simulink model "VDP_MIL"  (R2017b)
settings: Solver=FixedStepDiscrete  StartTime=0.0  StopTime=10.0  FixedStep=0.01  RelTol=1e-3  EnableMultiTasking=on
undefined symbols (not defined in the file): ASWTYPE_FALSE, ASWTYPE_TRUE, CcVDP_DiagPermitDelayTi_ms, CcVDP_Kl30VoltNorm2Over_mV, CcVDP_Kl30VoltNorm2Under_mV, CcVDP_Kl30VoltOver2Norm_mV, CcVDP_Kl30VoltUnder2Norm_mV, CcVDP_LeadAcidChgHvOnTi_ms, VDP0B5_RUNTIME_MS, VDP2A3_RUNTIME_MS, VDP_CONST2080_NUMB
libraries: AIWAYS_Powertrain_BMS_lib x36

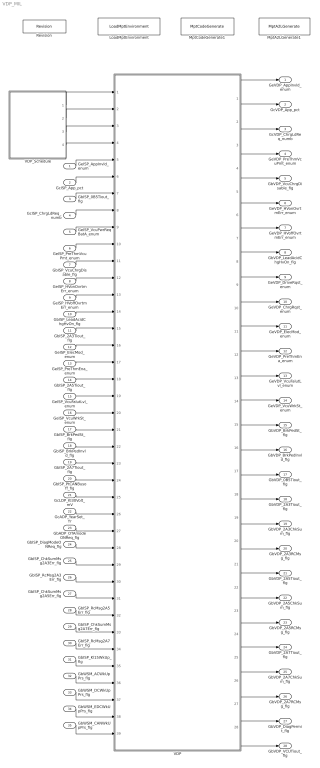
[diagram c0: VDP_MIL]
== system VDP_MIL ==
  GeISP_AppInvld_enum : Inport
  GcISP_App_pct : Inport  Port=2
  GbISP_0B5Tiout_flg : Inport  Port=3
  GcISP_ChrgLdReq_numb : Inport  Port=4
  GeISP_VcuPwrReqBatA_enum : Inport  Port=5
  GeISP_PreThmVcuPmt_enum : Inport  Port=6
  GbISP_VcuChrgDisable_flg : Inport  Port=7
  GeISP_HVonOvrtmErr_enum : Inport  Port=8
  GeISP_HVoffOvrtmErr_enum : Inport  Port=9
  GbISP_LeadAcidChgHvOn_flg : Inport  Port=10
  GbISP_2A3Tiout_flg : Inport  Port=11
  GeISP_ElecMod_enum : Inport  Port=12
  GeISP_PreThmEna_enum : Inport  Port=13
  GbISP_2A5Tiout_flg : Inport  Port=14
  GeISP_VcuFalutLvl_enum : Inport  Port=15
  GeISP_VcuWrkSt_enum : Inport  Port=16
  GbISP_BrkPedSt_flg : Inport  Port=17
  GbISP_BrkPedInvld_flg : Inport  Port=18
  GbISP_2A7Tiout_flg : Inport  Port=19
  GbISP_PtCANBusoff_flg : Inport  Port=20
  GcLDP_Kl30Volt_mV : Inport  Port=21
  GcADP_YearSet_Yr : Inport  Port=22
  GbADP_OTAmodeONReq_flg : Inport  Port=23
  GbISP_DiagModeONReq_flg : Inport  Port=24
  GbISP_ChkSumMsg2A3Err_flg : Inport  Port=25
  GbISP_RcMsg2A3Err_flg : Inport  Port=26
  GbISP_ChkSumMsg2A5Err_flg : Inport  Port=27
  GbISP_RcMsg2A5Err_flg : Inport  Port=28
  GbISP_ChkSumMsg2A7Err_flg : Inport  Port=29
  GbISP_RcMsg2A7Err_flg : Inport  Port=30
  GbISP_Kl15WkUp_flg : Inport  Port=31
  GbWSM_ACWkUpPrs_flg : Inport  Port=32
  GbWSM_DCWkUpPrs_flg : Inport  Port=33
  GbWSM_EDCWkUpPrs_flg : Inport  Port=34
  GbWSM_CANWkUpPrs_flg : Inport  Port=35
  LoadMptEnvironment : AIWAYS_Powertrain_BMS_lib/Config/LoadMptEnvironment  ProjectName=Comm  SuppierID=NewPlatformUAES
  MptA2LGenerate1 : AIWAYS_Powertrain_BMS_lib/Config/MptA2LGenerate  SystemSampleTime=-1
  MptCodeGenerate1 : AIWAYS_Powertrain_BMS_lib/Config/MptCodeGenerate  SystemSampleTime=-1
  Revision : AIWAYS_Powertrain_BMS_lib/Config/Revision  curVersion='M107C106'  newVersion='M107C106'
  VDP : Subsystem
  VDP_Schedule : Stateflow chart  TreatAsAtomicUnit=on
  GeVDP_AppInvld_enum : Outport
  GcVDP_App_pct : Outport  Port=2
  GcVDP_ChrgLdReq_numb : Outport  Port=3
  GeVDP_PreThmVcuPmt_enum : Outport  Port=4
  GbVDP_VcuChrgDisable_flg : Outport  Port=5
  GeVDP_HVonOvrtmErr_enum : Outport  Port=6
  GeVDP_HVoffOvrtmErr_enum : Outport  Port=7
  GbVDP_LeadAcidChgHvOn_flg : Outport  Port=8
  GeVDP_DriveRqst_enum : Outport  Port=9
  GeVDP_ChrgRqst_enum : Outport  Port=10
  GeVDP_ElecMod_enum : Outport  Port=11
  GeVDP_PreThmEna_enum : Outport  Port=12
  GeVDP_VcuFalutLvl_enum : Outport  Port=13
  GeVDP_VcuWrkSt_enum : Outport  Port=14
  GbVDP_BrkPedSt_flg : Outport  Port=15
  GbVDP_BrkPedInvld_flg : Outport  Port=16
  GbVDP_0B5Tiout_flg : Outport  Port=17
  GbVDP_2A3Tiout_flg : Outport  Port=18
  GbVDP_2A3ChkSum_flg : Outport  Port=19
  GbVDP_2A3RCMsg_flg : Outport  Port=20
  GbVDP_2A5Tiout_flg : Outport  Port=21
  GbVDP_2A5ChkSum_flg : Outport  Port=22
  GbVDP_2A5RCMsg_flg : Outport  Port=23
  GbVDP_2A7Tiout_flg : Outport  Port=24
  GbVDP_2A7ChkSum_flg : Outport  Port=25
  GbVDP_2A7RCMsg_flg : Outport  Port=26
  GbVDP_DiagPermit_flg : Outport  Port=27
  GbVDP_VCUTiout_flg : Outport  Port=28
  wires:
  GeISP_AppInvld_enum/1 -> VDP/5(GeISP_AppInvld_enum)
  GcISP_App_pct/1 -> VDP/6(GcISP_App_pct)
  GbISP_0B5Tiout_flg/1 -> VDP/7(GbISP_0B5Tiout_flg)
  GcISP_ChrgLdReq_numb/1 -> VDP/8(GcISP_ChrgLdReq_numb)
  GeISP_VcuPwrReqBatA_enum/1 -> VDP/9(GeISP_VcuPwrReqBatA_enum)
  GeISP_PreThmVcuPmt_enum/1 -> VDP/10(GeISP_PreThmVcuPmt_enum)
  GbISP_VcuChrgDisable_flg/1 -> VDP/11(GbISP_VcuChrgDisable_flg)
  GeISP_HVonOvrtmErr_enum/1 -> VDP/12(GeISP_HVonOvrtmErr_enum)
  GeISP_HVoffOvrtmErr_enum/1 -> VDP/13(GeISP_HVoffOvrtmErr_enum)
  GbISP_LeadAcidChgHvOn_flg/1 -> VDP/14(GbISP_LeadAcidChgHvOn_flg)
  GbISP_2A3Tiout_flg/1 -> VDP/15(GbISP_2A3Tiout_flg)
  GeISP_ElecMod_enum/1 -> VDP/16(GeISP_ElecMod_enum)
  GeISP_PreThmEna_enum/1 -> VDP/17(GeISP_PreThmEna_enum)
  GbISP_2A5Tiout_flg/1 -> VDP/18(GbISP_2A5Tiout_flg)
  GeISP_VcuFalutLvl_enum/1 -> VDP/19(GeISP_VcuFalutLvl_enum)
  GeISP_VcuWrkSt_enum/1 -> VDP/20(GeISP_VcuWrkSt_enum)
  GbISP_BrkPedSt_flg/1 -> VDP/21(GbISP_BrkPedSt_flg)
  GbISP_BrkPedInvld_flg/1 -> VDP/22(GbISP_BrkPedInvld_flg)
  GbISP_2A7Tiout_flg/1 -> VDP/23(GbISP_2A7Tiout_flg)
  VDP/1(GeVDP_AppInvld_enum) -> GeVDP_AppInvld_enum/1
  VDP/2(GcVDP_App_pct) -> GcVDP_App_pct/1
  VDP/3(GcVDP_ChrgLdReq_numb) -> GcVDP_ChrgLdReq_numb/1
  VDP/4(GeVDP_PreThmVcuPmt_enum) -> GeVDP_PreThmVcuPmt_enum/1
  VDP/5(GbVDP_VcuChrgDisable_flg) -> GbVDP_VcuChrgDisable_flg/1
  VDP/6(GeVDP_HVonOvrtmErr_enum) -> GeVDP_HVonOvrtmErr_enum/1
  VDP/7(GeVDP_HVoffOvrtmErr_enum) -> GeVDP_HVoffOvrtmErr_enum/1
  VDP/8(GbVDP_LeadAcidChgHvOn_flg) -> GbVDP_LeadAcidChgHvOn_flg/1
  VDP/9(GeVDP_DriveRqst_enum) -> GeVDP_DriveRqst_enum/1
  VDP/10(GeVDP_ChrgRqst_enum) -> GeVDP_ChrgRqst_enum/1
  VDP/11(GeVDP_ElecMod_enum) -> GeVDP_ElecMod_enum/1
  VDP/12(GeVDP_PreThmEna_enum) -> GeVDP_PreThmEna_enum/1
  VDP/13(GeVDP_VcuFalutLvl_enum) -> GeVDP_VcuFalutLvl_enum/1
  VDP/14(GeVDP_VcuWrkSt_enum) -> GeVDP_VcuWrkSt_enum/1
  VDP/15(GbVDP_BrkPedSt_flg) -> GbVDP_BrkPedSt_flg/1
  VDP/16(GbVDP_BrkPedInvld_flg) -> GbVDP_BrkPedInvld_flg/1
  GbISP_DiagModeONReq_flg/1 -> VDP/28(GbISP_DiagModeONReq_flg)
  GcLDP_Kl30Volt_mV/1 -> VDP/25(GcLDP_Kl30Volt_mV)
  GbADP_OTAmodeONReq_flg/1 -> VDP/27(GbADP_OTAmodeONReq_flg)
  GcADP_YearSet_Yr/1 -> VDP/26(GcADP_YearSet_Yr)
  GbISP_PtCANBusoff_flg/1 -> VDP/24(GbISP_PtCANBusoff_flg)
  GbISP_ChkSumMsg2A3Err_flg/1 -> VDP/29(GbISP_ChkSumMsg2A3Err_flg)
  GbISP_RcMsg2A3Err_flg/1 -> VDP/30(GbISP_RcMsg2A3Err_flg)
  GbISP_RcMsg2A5Err_flg/1 -> VDP/32(GbISP_RcMsg2A5Err_flg)
  GbISP_ChkSumMsg2A5Err_flg/1 -> VDP/31(GbISP_ChkSumMsg2A5Err_flg)
  GbISP_RcMsg2A7Err_flg/1 -> VDP/34(GbISP_RcMsg2A7Err_flg)
  GbISP_ChkSumMsg2A7Err_flg/1 -> VDP/33(GbISP_ChkSumMsg2A7Err_flg)
  VDP/17(GbVDP_0B5Tiout_flg) -> GbVDP_0B5Tiout_flg/1
  VDP/20(GbVDP_2A3RCMsg_flg) -> GbVDP_2A3RCMsg_flg/1
  VDP/18(GbVDP_2A3Tiout_flg) -> GbVDP_2A3Tiout_flg/1
  VDP/19(GbVDP_2A3ChkSum_flg) -> GbVDP_2A3ChkSum_flg/1
  VDP/23(GbVDP_2A5RCMsg_flg) -> GbVDP_2A5RCMsg_flg/1
  VDP/21(GbVDP_2A5Tiout_flg) -> GbVDP_2A5Tiout_flg/1
  VDP/22(GbVDP_2A5ChkSum_flg) -> GbVDP_2A5ChkSum_flg/1
  VDP/25(GbVDP_2A7ChkSum_flg) -> GbVDP_2A7ChkSum_flg/1
  VDP/24(GbVDP_2A7Tiout_flg) -> GbVDP_2A7Tiout_flg/1
  VDP/26(GbVDP_2A7RCMsg_flg) -> GbVDP_2A7RCMsg_flg/1
  VDP/27(GbVDP_DiagPermit_flg) -> GbVDP_DiagPermit_flg/1
  VDP/28(GbVDP_VCUTiout_flg) -> GbVDP_VCUTiout_flg/1
  GbISP_Kl15WkUp_flg/1 -> VDP/35(GbISP_Kl15WkUp_flg)
  GbWSM_ACWkUpPrs_flg/1 -> VDP/36(GbWSM_ACWkUpPrs_flg)
  GbWSM_CANWkUpPrs_flg/1 -> VDP/39(GbWSM_CANWkUpPrs_flg)
  GbWSM_EDCWkUpPrs_flg/1 -> VDP/38(GbWSM_EDCWkUpPrs_flg)
  GbWSM_DCWkUpPrs_flg/1 -> VDP/37(GbWSM_DCWkUpPrs_flg)
  VDP_Schedule/1(VDP_0B5_10ms()) -> VDP/1(VDP_0B5_10ms)
  VDP_Schedule/2(VDP_2A3_10ms()) -> VDP/2(VDP_2A3_10ms)
  VDP_Schedule/3(VDP_2A5_100ms()) -> VDP/3(VDP_2A5_100ms)
  VDP_Schedule/4(VDP_2A7_100ms()) -> VDP/4(VDP_2A7_100ms)

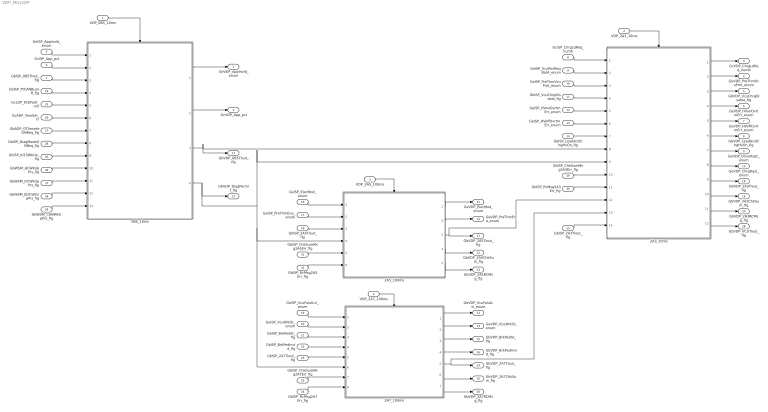
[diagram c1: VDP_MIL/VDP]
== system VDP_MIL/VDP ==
  VDP_0B5_10ms : Inport
  VDP_2A3_10ms : Inport  Port=2
  VDP_2A5_100ms : Inport  Port=3
  VDP_2A7_100ms : Inport  Port=4
  GeISP_AppInvld_enum : Inport  Port=5
  GcISP_App_pct : Inport  Port=6
  GbISP_0B5Tiout_flg : Inport  Port=7
  GcISP_ChrgLdReq_numb : Inport  Port=8
  GeISP_VcuPwrReqBatA_enum : Inport  Port=9
  GeISP_PreThmVcuPmt_enum : Inport  Port=10
  GbISP_VcuChrgDisable_flg : Inport  Port=11
  GeISP_HVonOvrtmErr_enum : Inport  Port=12
  GeISP_HVoffOvrtmErr_enum : Inport  Port=13
  GbISP_LeadAcidChgHvOn_flg : Inport  Port=14
  GbISP_2A3Tiout_flg : Inport  Port=15
  GeISP_ElecMod_enum : Inport  Port=16
  GeISP_PreThmEna_enum : Inport  Port=17
  GbISP_2A5Tiout_flg : Inport  Port=18
  GeISP_VcuFalutLvl_enum : Inport  Port=19
  GeISP_VcuWrkSt_enum : Inport  Port=20
  GbISP_BrkPedSt_flg : Inport  Port=21
  GbISP_BrkPedInvld_flg : Inport  Port=22
  GbISP_2A7Tiout_flg : Inport  Port=23
  GbISP_PtCANBusoff_flg : Inport  Port=24
  GcLDP_Kl30Volt_mV : Inport  Port=25
  GcADP_YearSet_Yr : Inport  Port=26
  GbADP_OTAmodeONReq_flg : Inport  Port=27
  GbISP_DiagModeONReq_flg : Inport  Port=28
  GbISP_ChkSumMsg2A3Err_flg : Inport  Port=29
  GbISP_RcMsg2A3Err_flg : Inport  Port=30
  GbISP_ChkSumMsg2A5Err_flg : Inport  Port=31
  GbISP_RcMsg2A5Err_flg : Inport  Port=32
  GbISP_ChkSumMsg2A7Err_flg : Inport  Port=33
  GbISP_RcMsg2A7Err_flg : Inport  Port=34
  GbISP_Kl15WkUp_flg : Inport  Port=35
  GbWSM_ACWkUpPrs_flg : Inport  Port=36
  GbWSM_DCWkUpPrs_flg : Inport  Port=37
  GbWSM_EDCWkUpPrs_flg : Inport  Port=38
  GbWSM_CANWkUpPrs_flg : Inport  Port=39
  0B5_10ms : Subsystem
  2A3_10ms : Subsystem
  2A5_100ms : Subsystem
  2A7_100ms : Subsystem
  GeVDP_AppInvld_enum : Outport
  GcVDP_App_pct : Outport  Port=2
  GcVDP_ChrgLdReq_numb : Outport  Port=3
  GeVDP_PreThmVcuPmt_enum : Outport  Port=4
  GbVDP_VcuChrgDisable_flg : Outport  Port=5
  GeVDP_HVonOvrtmErr_enum : Outport  Port=6
  GeVDP_HVoffOvrtmErr_enum : Outport  Port=7
  GbVDP_LeadAcidChgHvOn_flg : Outport  Port=8
  GeVDP_DriveRqst_enum : Outport  Port=9
  GeVDP_ChrgRqst_enum : Outport  Port=10
  GeVDP_ElecMod_enum : Outport  Port=11
  GeVDP_PreThmEna_enum : Outport  Port=12
  GeVDP_VcuFalutLvl_enum : Outport  Port=13
  GeVDP_VcuWrkSt_enum : Outport  Port=14
  GbVDP_BrkPedSt_flg : Outport  Port=15
  GbVDP_BrkPedInvld_flg : Outport  Port=16
  GbVDP_0B5Tiout_flg : Outport  Port=17
  GbVDP_2A3Tiout_flg : Outport  Port=18
  GbVDP_2A3ChkSum_flg : Outport  Port=19
  GbVDP_2A3RCMsg_flg : Outport  Port=20
  GbVDP_2A5Tiout_flg : Outport  Port=21
  GbVDP_2A5ChkSum_flg : Outport  Port=22
  GbVDP_2A5RCMsg_flg : Outport  Port=23
  GbVDP_2A7Tiout_flg : Outport  Port=24
  GbVDP_2A7ChkSum_flg : Outport  Port=25
  GbVDP_2A7RCMsg_flg : Outport  Port=26
  GbVDP_DiagPermit_flg : Outport  Port=27
  GbVDP_VCUTiout_flg : Outport  Port=28
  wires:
  VDP_2A3_10ms/1 -> 2A3_10ms/Trigger
  VDP_2A5_100ms/1 -> 2A5_100ms/Trigger
  VDP_2A7_100ms/1 -> 2A7_100ms/Trigger
  GeISP_AppInvld_enum/1 -> 0B5_10ms/1(GeISP_AppInvld_enum)
  GcISP_App_pct/1 -> 0B5_10ms/2(GcISP_App_pct)
  GbISP_0B5Tiout_flg/1 -> 0B5_10ms/3(GbISP_0B5Tiout_flg)
  0B5_10ms/1(GeVDP_AppInvld_enum) -> GeVDP_AppInvld_enum/1
  0B5_10ms/2(GcVDP_App_pct) -> GcVDP_App_pct/1
  GcISP_ChrgLdReq_numb/1 -> 2A3_10ms/1(GcISP_ChrgLdReq_numb)
  GeISP_VcuPwrReqBatA_enum/1 -> 2A3_10ms/2(GeISP_VcuPwrReqBatA_enum)
  GeISP_PreThmVcuPmt_enum/1 -> 2A3_10ms/3(GeISP_PreThmVcuPmt_enum)
  GbISP_VcuChrgDisable_flg/1 -> 2A3_10ms/4(GbISP_VcuChrgDisable_flg)
  GeISP_HVonOvrtmErr_enum/1 -> 2A3_10ms/5(GeISP_HVonOvrtmErr_enum)
  GeISP_HVoffOvrtmErr_enum/1 -> 2A3_10ms/6(GeISP_HVoffOvrtmErr_enum)
  GbISP_LeadAcidChgHvOn_flg/1 -> 2A3_10ms/7(GbISP_LeadAcidChgHvOn_flg)
  GbISP_2A3Tiout_flg/1 -> 2A3_10ms/14(GbISP_2A3Tiout_flg)
  2A3_10ms/5(GeVDP_HVoffOvrtmErr_enum) -> GeVDP_HVoffOvrtmErr_enum/1
  2A3_10ms/4(GeVDP_HVonOvrtmErr_enum) -> GeVDP_HVonOvrtmErr_enum/1
  2A3_10ms/6(GbVDP_LeadAcidChgHvOn_flg) -> GbVDP_LeadAcidChgHvOn_flg/1
  2A3_10ms/3(GbVDP_VcuChrgDisable_flg) -> GbVDP_VcuChrgDisable_flg/1
  2A3_10ms/2(GeVDP_PreThmVcuPmt_enum) -> GeVDP_PreThmVcuPmt_enum/1
  2A3_10ms/1(GcVDP_ChrgLdReq_numb) -> GcVDP_ChrgLdReq_numb/1
  2A3_10ms/7(GeVDP_DriveRqst_enum) -> GeVDP_DriveRqst_enum/1
  2A3_10ms/8(GeVDP_ChrgRqst_enum) -> GeVDP_ChrgRqst_enum/1
  GeISP_ElecMod_enum/1 -> 2A5_100ms/1(GeISP_ElecMod_enum)
  GeISP_PreThmEna_enum/1 -> 2A5_100ms/2(GeISP_PreThmEna_enum)
  GbISP_2A5Tiout_flg/1 -> 2A5_100ms/3(GbISP_2A5Tiout_flg)
  2A5_100ms/1(GeVDP_ElecMod_enum) -> GeVDP_ElecMod_enum/1
  2A5_100ms/2(GeVDP_PreThmEna_enum) -> GeVDP_PreThmEna_enum/1
  GeISP_VcuFalutLvl_enum/1 -> 2A7_100ms/1(GeISP_VcuFalutLvl_enum)
  GeISP_VcuWrkSt_enum/1 -> 2A7_100ms/2(GeISP_VcuWrkSt_enum)
  GbISP_BrkPedSt_flg/1 -> 2A7_100ms/3(GbISP_BrkPedSt_flg)
  GbISP_BrkPedInvld_flg/1 -> 2A7_100ms/4(GbISP_BrkPedInvld_flg)
  GbISP_2A7Tiout_flg/1 -> 2A7_100ms/5(GbISP_2A7Tiout_flg)
  2A7_100ms/1(GeVDP_VcuFalutLvl_enum) -> GeVDP_VcuFalutLvl_enum/1
  2A7_100ms/2(GeVDP_VcuWrkSt_enum) -> GeVDP_VcuWrkSt_enum/1
  2A7_100ms/3(GbVDP_BrkPedSt_flg) -> GbVDP_BrkPedSt_flg/1
  2A7_100ms/4(GbVDP_BrkPedInvld_flg) -> GbVDP_BrkPedInvld_flg/1
  0B5_10ms/3(GbVDP_0B5Tiout_flg) -> GbVDP_0B5Tiout_flg/1, 2A3_10ms/8(GbVDP_0B5Tiout_flg)
  GbISP_ChkSumMsg2A3Err_flg/1 -> 2A3_10ms/10(GbISP_ChkSumMsg2A3Err_flg)
  GbISP_RcMsg2A3Err_flg/1 -> 2A3_10ms/11(GbISP_RcMsg2A3Err_flg)
  2A3_10ms/9(GbVDP_2A3Tiout_flg) -> GbVDP_2A3Tiout_flg/1
  2A3_10ms/10(GbVDP_2A3ChkSum_flg) -> GbVDP_2A3ChkSum_flg/1
  2A3_10ms/11(GbVDP_2A3RCMsg_flg) -> GbVDP_2A3RCMsg_flg/1
  GbISP_ChkSumMsg2A5Err_flg/1 -> 2A5_100ms/5(GbISP_ChkSumMsg2A5Err_flg)
  GbISP_RcMsg2A5Err_flg/1 -> 2A5_100ms/6(GbISP_RcMsg2A5Err_flg)
  2A5_100ms/5(GbVDP_2A5RCMsg_flg) -> GbVDP_2A5RCMsg_flg/1
  2A5_100ms/3(GbVDP_2A5Tiout_flg) -> GbVDP_2A5Tiout_flg/1, 2A3_10ms/12(GbVDP_2A5Tiout_flg)
  2A5_100ms/4(GbVDP_2A5ChkSum_flg) -> GbVDP_2A5ChkSum_flg/1
  GbISP_RcMsg2A7Err_flg/1 -> 2A7_100ms/8(GbISP_RcMsg2A7Err_flg)
  GbISP_ChkSumMsg2A7Err_flg/1 -> 2A7_100ms/7(GbISP_ChkSumMsg2A7Err_flg)
  2A7_100ms/7(GbVDP_2A7RCMsg_flg) -> GbVDP_2A7RCMsg_flg/1
  2A7_100ms/5(GbVDP_2A7Tiout_flg) -> GbVDP_2A7Tiout_flg/1, 2A3_10ms/13(GbVDP_2A7Tiout_flg)
  2A7_100ms/6(GbVDP_2A7ChkSum_flg) -> GbVDP_2A7ChkSum_flg/1
  GcLDP_Kl30Volt_mV/1 -> 0B5_10ms/5(GcLDP_Kl30Volt_mV)
  GcADP_YearSet_Yr/1 -> 0B5_10ms/6(GcADP_YearSet_Yr)
  GbADP_OTAmodeONReq_flg/1 -> 0B5_10ms/7(GbADP_OTAmodeONReq_flg)
  GbISP_DiagModeONReq_flg/1 -> 0B5_10ms/8(GbISP_DiagModeONReq_flg)
  0B5_10ms/4(GbVDP_DiagPermit_flg) -> 2A7_100ms/6(GbVDP_DiagPermit_flg), 2A5_100ms/4(GbVDP_DiagPermit_flg), 2A3_10ms/9(GbVDP_DiagPermit_flg), GbVDP_DiagPermit_flg/1
  VDP_0B5_10ms/1 -> 0B5_10ms/Trigger
  GbISP_PtCANBusoff_flg/1 -> 0B5_10ms/4(GbISP_PtCANBusoff_flg)
  2A3_10ms/12(GbVDP_VCUTiout_flg) -> GbVDP_VCUTiout_flg/1
  GbISP_Kl15WkUp_flg/1 -> 0B5_10ms/9(GbISP_Kl15WkUp_flg)
  GbWSM_CANWkUpPrs_flg/1 -> 0B5_10ms/13(GbWSM_CANWkUpPrs_flg)
  GbWSM_EDCWkUpPrs_flg/1 -> 0B5_10ms/12(GbWSM_EDCWkUpPrs_flg)
  GbWSM_DCWkUpPrs_flg/1 -> 0B5_10ms/11(GbWSM_DCWkUpPrs_flg)
  GbWSM_ACWkUpPrs_flg/1 -> 0B5_10ms/10(GbWSM_ACWkUpPrs_flg)

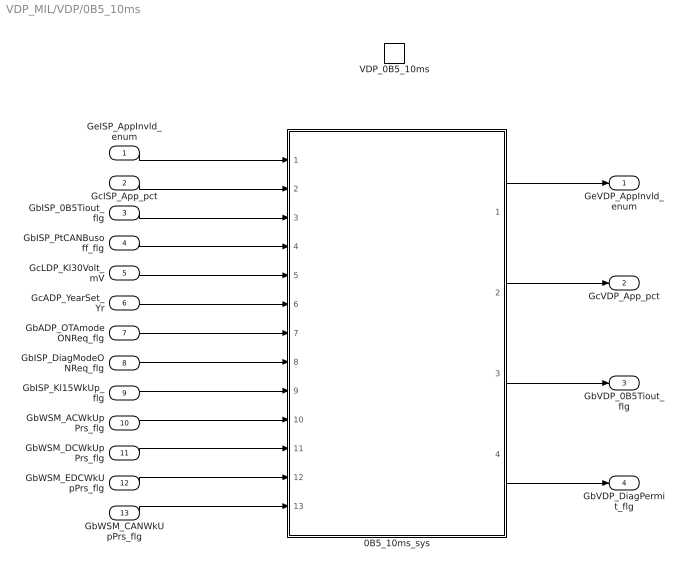
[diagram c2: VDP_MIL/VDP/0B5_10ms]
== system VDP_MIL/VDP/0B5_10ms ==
  GeISP_AppInvld_enum : Inport
  GcISP_App_pct : Inport  Port=2
  GbISP_0B5Tiout_flg : Inport  Port=3
  GbISP_PtCANBusoff_flg : Inport  Port=4
  GcLDP_Kl30Volt_mV : Inport  Port=5
  GcADP_YearSet_Yr : Inport  Port=6
  GbADP_OTAmodeONReq_flg : Inport  Port=7
  GbISP_DiagModeONReq_flg : Inport  Port=8
  GbISP_Kl15WkUp_flg : Inport  Port=9
  GbWSM_ACWkUpPrs_flg : Inport  Port=10
  GbWSM_DCWkUpPrs_flg : Inport  Port=11
  GbWSM_EDCWkUpPrs_flg : Inport  Port=12
  GbWSM_CANWkUpPrs_flg : Inport  Port=13
  VDP_0B5_10ms : TriggerPort  TriggerType=function-call  VariantControl=(inherit)
  0B5_10ms_sys : Subsystem
  GeVDP_AppInvld_enum : Outport
  GcVDP_App_pct : Outport  Port=2
  GbVDP_0B5Tiout_flg : Outport  Port=3
  GbVDP_DiagPermit_flg : Outport  Port=4
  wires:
  GeISP_AppInvld_enum/1 -> 0B5_10ms_sys/1(GeISP_AppInvld_enum)
  GcISP_App_pct/1 -> 0B5_10ms_sys/2(GcISP_App_pct)
  GbISP_0B5Tiout_flg/1 -> 0B5_10ms_sys/3(GbISP_0B5Tiout_flg)
  0B5_10ms_sys/1(GeVDP_AppInvld_enum) -> GeVDP_AppInvld_enum/1
  0B5_10ms_sys/2(GcVDP_App_pct) -> GcVDP_App_pct/1
  0B5_10ms_sys/3(GbVDP_0B5Tiout_flg) -> GbVDP_0B5Tiout_flg/1
  GbISP_PtCANBusoff_flg/1 -> 0B5_10ms_sys/4(GbISP_PtCANBusoff_flg)
  GbISP_DiagModeONReq_flg/1 -> 0B5_10ms_sys/8(GbISP_DiagModeONReq_flg)
  GcADP_YearSet_Yr/1 -> 0B5_10ms_sys/6(GcADP_YearSet_Yr)
  GcLDP_Kl30Volt_mV/1 -> 0B5_10ms_sys/5(GcLDP_Kl30Volt_mV)
  GbADP_OTAmodeONReq_flg/1 -> 0B5_10ms_sys/7(GbADP_OTAmodeONReq_flg)
  0B5_10ms_sys/4(GbVDP_DiagPermit_flg) -> GbVDP_DiagPermit_flg/1
  GbISP_Kl15WkUp_flg/1 -> 0B5_10ms_sys/9(GbWSM_Kl15WkUpPrs_flg)
  GbWSM_ACWkUpPrs_flg/1 -> 0B5_10ms_sys/10(GbWSM_ACWkUpPrs_flg)
  GbWSM_DCWkUpPrs_flg/1 -> 0B5_10ms_sys/11(GbWSM_DCWkUpPrs_flg)
  GbWSM_EDCWkUpPrs_flg/1 -> 0B5_10ms_sys/12(GbWSM_EDCWkUpPrs_flg)
  GbWSM_CANWkUpPrs_flg/1 -> 0B5_10ms_sys/13(GbWSM_CANWkUpPrs_flg)

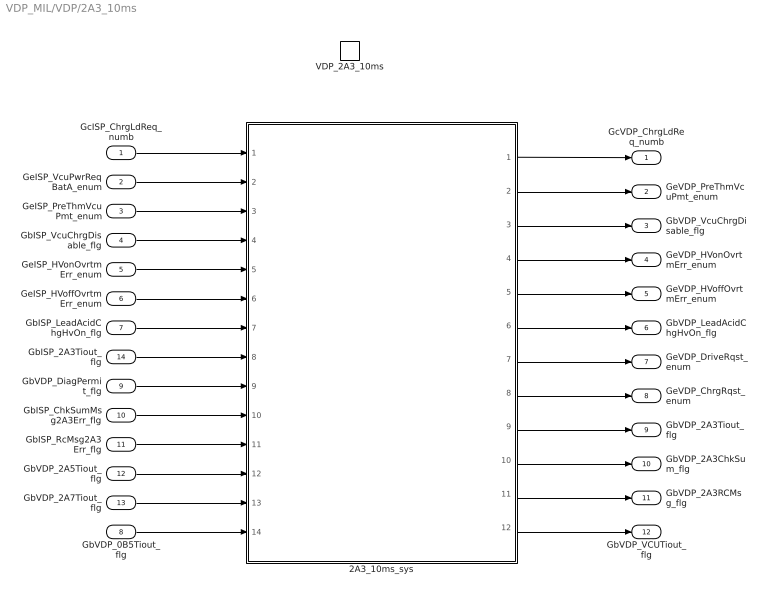
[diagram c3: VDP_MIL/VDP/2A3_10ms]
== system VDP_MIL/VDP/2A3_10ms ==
  GcISP_ChrgLdReq_numb : Inport
  GeISP_VcuPwrReqBatA_enum : Inport  Port=2
  GeISP_PreThmVcuPmt_enum : Inport  Port=3
  GbISP_VcuChrgDisable_flg : Inport  Port=4
  GeISP_HVonOvrtmErr_enum : Inport  Port=5
  GeISP_HVoffOvrtmErr_enum : Inport  Port=6
  GbISP_LeadAcidChgHvOn_flg : Inport  Port=7
  GbVDP_0B5Tiout_flg : Inport  Port=8
  GbVDP_DiagPermit_flg : Inport  Port=9
  GbISP_ChkSumMsg2A3Err_flg : Inport  Port=10
  GbISP_RcMsg2A3Err_flg : Inport  Port=11
  GbVDP_2A5Tiout_flg : Inport  Port=12
  GbVDP_2A7Tiout_flg : Inport  Port=13
  GbISP_2A3Tiout_flg : Inport  Port=14
  VDP_2A3_10ms : TriggerPort  TriggerType=function-call  VariantControl=(inherit)
  2A3_10ms_sys : Subsystem
  GcVDP_ChrgLdReq_numb : Outport
  GeVDP_PreThmVcuPmt_enum : Outport  Port=2
  GbVDP_VcuChrgDisable_flg : Outport  Port=3
  GeVDP_HVonOvrtmErr_enum : Outport  Port=4
  GeVDP_HVoffOvrtmErr_enum : Outport  Port=5
  GbVDP_LeadAcidChgHvOn_flg : Outport  Port=6
  GeVDP_DriveRqst_enum : Outport  Port=7
  GeVDP_ChrgRqst_enum : Outport  Port=8
  GbVDP_2A3Tiout_flg : Outport  Port=9
  GbVDP_2A3ChkSum_flg : Outport  Port=10
  GbVDP_2A3RCMsg_flg : Outport  Port=11
  GbVDP_VCUTiout_flg : Outport  Port=12
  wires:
  GcISP_ChrgLdReq_numb/1 -> 2A3_10ms_sys/1(GcISP_ChrgLdReq_numb)
  GeISP_VcuPwrReqBatA_enum/1 -> 2A3_10ms_sys/2(GeISP_VcuPwrReqBatA_enum)
  GeISP_PreThmVcuPmt_enum/1 -> 2A3_10ms_sys/3(GeISP_PreThmVcuPmt_enum)
  GbISP_VcuChrgDisable_flg/1 -> 2A3_10ms_sys/4(GbISP_VcuChrgDisable_flg)
  GeISP_HVonOvrtmErr_enum/1 -> 2A3_10ms_sys/5(GeISP_HVonOvrtmErr_enum)
  GeISP_HVoffOvrtmErr_enum/1 -> 2A3_10ms_sys/6(GeISP_HVoffOvrtmErr_enum)
  GbISP_LeadAcidChgHvOn_flg/1 -> 2A3_10ms_sys/7(GbISP_LeadAcidChgHvOn_flg)
  GbISP_2A3Tiout_flg/1 -> 2A3_10ms_sys/8(GbISP_2A3Tiout_flg)
  2A3_10ms_sys/1(GcVDP_ChrgLdReq_numb) -> GcVDP_ChrgLdReq_numb/1
  2A3_10ms_sys/2(GeVDP_PreThmVcuPmt_enum) -> GeVDP_PreThmVcuPmt_enum/1
  2A3_10ms_sys/3(GbVDP_VcuChrgDisable_flg) -> GbVDP_VcuChrgDisable_flg/1
  2A3_10ms_sys/4(GeVDP_HVonOvrtmErr_enum) -> GeVDP_HVonOvrtmErr_enum/1
  2A3_10ms_sys/5(GeVDP_HVoffOvrtmErr_enum) -> GeVDP_HVoffOvrtmErr_enum/1
  2A3_10ms_sys/6(GbVDP_LeadAcidChgHvOn_flg) -> GbVDP_LeadAcidChgHvOn_flg/1
  2A3_10ms_sys/7(GeVDP_DriveRqst_enum) -> GeVDP_DriveRqst_enum/1
  2A3_10ms_sys/8(GeVDP_ChrgRqst_enum) -> GeVDP_ChrgRqst_enum/1
  GbVDP_DiagPermit_flg/1 -> 2A3_10ms_sys/9(GbVDP_DiagPermit_flg)
  2A3_10ms_sys/9(GbVDP_2A3Tiout_flg) -> GbVDP_2A3Tiout_flg/1
  2A3_10ms_sys/10(GbVDP_2A3ChkSum_flg) -> GbVDP_2A3ChkSum_flg/1
  2A3_10ms_sys/11(GbVDP_2A3RCMsg_flg) -> GbVDP_2A3RCMsg_flg/1
  GbISP_ChkSumMsg2A3Err_flg/1 -> 2A3_10ms_sys/10(GbISP_ChkSumMsg2A3Err_flg)
  GbISP_RcMsg2A3Err_flg/1 -> 2A3_10ms_sys/11(GbISP_RcMsg2A3Err_flg)
  2A3_10ms_sys/12(GbVDP_VCUTiout_flg) -> GbVDP_VCUTiout_flg/1
  GbVDP_2A5Tiout_flg/1 -> 2A3_10ms_sys/12(GbVDP_2A5Tiout_flg)
  GbVDP_2A7Tiout_flg/1 -> 2A3_10ms_sys/13(GbVDP_2A7Tiout_flg)
  GbVDP_0B5Tiout_flg/1 -> 2A3_10ms_sys/14(GbVDP_0B5Tiout_flg)

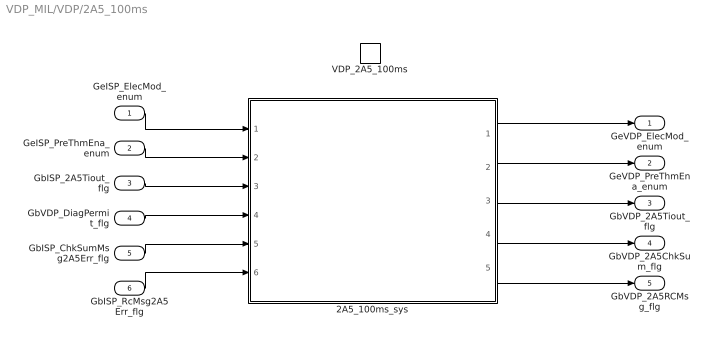
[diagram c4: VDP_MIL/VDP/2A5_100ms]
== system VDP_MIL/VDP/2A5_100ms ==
  GeISP_ElecMod_enum : Inport
  GeISP_PreThmEna_enum : Inport  Port=2
  GbISP_2A5Tiout_flg : Inport  Port=3
  GbVDP_DiagPermit_flg : Inport  Port=4
  GbISP_ChkSumMsg2A5Err_flg : Inport  Port=5
  GbISP_RcMsg2A5Err_flg : Inport  Port=6
  VDP_2A5_100ms : TriggerPort  TriggerType=function-call  VariantControl=(inherit)
  2A5_100ms_sys : Subsystem
  GeVDP_ElecMod_enum : Outport
  GeVDP_PreThmEna_enum : Outport  Port=2
  GbVDP_2A5Tiout_flg : Outport  Port=3
  GbVDP_2A5ChkSum_flg : Outport  Port=4
  GbVDP_2A5RCMsg_flg : Outport  Port=5
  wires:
  GeISP_ElecMod_enum/1 -> 2A5_100ms_sys/1(GeISP_ElecMod_enum)
  GeISP_PreThmEna_enum/1 -> 2A5_100ms_sys/2(GeISP_PreThmEna_enum)
  GbISP_2A5Tiout_flg/1 -> 2A5_100ms_sys/3(GbISP_2A5Tiout_flg)
  2A5_100ms_sys/1(GeVDP_ElecMod_enum) -> GeVDP_ElecMod_enum/1
  2A5_100ms_sys/2(GeVDP_PreThmEna_enum) -> GeVDP_PreThmEna_enum/1
  GbVDP_DiagPermit_flg/1 -> 2A5_100ms_sys/4(GbVDP_DiagPermit_flg)
  2A5_100ms_sys/3(GbVDP_2A5Tiout_flg) -> GbVDP_2A5Tiout_flg/1
  2A5_100ms_sys/4(GbVDP_2A5ChkSum_flg) -> GbVDP_2A5ChkSum_flg/1
  2A5_100ms_sys/5(GbVDP_2A5RCMsg_flg) -> GbVDP_2A5RCMsg_flg/1
  GbISP_ChkSumMsg2A5Err_flg/1 -> 2A5_100ms_sys/5(GbISP_ChkSumMsg2A5Err_flg)
  GbISP_RcMsg2A5Err_flg/1 -> 2A5_100ms_sys/6(GbISP_RcMsg2A5Err_flg)

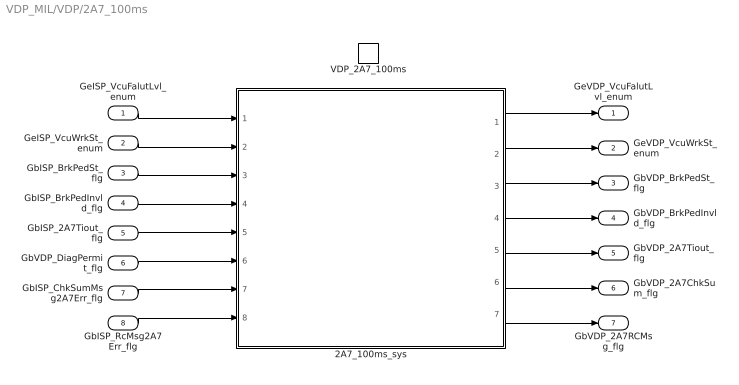
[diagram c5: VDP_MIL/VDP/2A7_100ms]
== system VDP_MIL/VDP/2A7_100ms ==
  GeISP_VcuFalutLvl_enum : Inport
  GeISP_VcuWrkSt_enum : Inport  Port=2
  GbISP_BrkPedSt_flg : Inport  Port=3
  GbISP_BrkPedInvld_flg : Inport  Port=4
  GbISP_2A7Tiout_flg : Inport  Port=5
  GbVDP_DiagPermit_flg : Inport  Port=6
  GbISP_ChkSumMsg2A7Err_flg : Inport  Port=7
  GbISP_RcMsg2A7Err_flg : Inport  Port=8
  VDP_2A7_100ms : TriggerPort  TriggerType=function-call  VariantControl=(inherit)
  2A7_100ms_sys : Subsystem
  GeVDP_VcuFalutLvl_enum : Outport
  GeVDP_VcuWrkSt_enum : Outport  Port=2
  GbVDP_BrkPedSt_flg : Outport  Port=3
  GbVDP_BrkPedInvld_flg : Outport  Port=4
  GbVDP_2A7Tiout_flg : Outport  Port=5
  GbVDP_2A7ChkSum_flg : Outport  Port=6
  GbVDP_2A7RCMsg_flg : Outport  Port=7
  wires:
  GeISP_VcuFalutLvl_enum/1 -> 2A7_100ms_sys/1(GeISP_VcuFalutLvl_enum)
  GeISP_VcuWrkSt_enum/1 -> 2A7_100ms_sys/2(GeISP_VcuWrkSt_enum)
  GbISP_BrkPedSt_flg/1 -> 2A7_100ms_sys/3(GbISP_BrkPedSt_flg)
  GbISP_BrkPedInvld_flg/1 -> 2A7_100ms_sys/4(GbISP_BrkPedInvld_flg)
  GbISP_2A7Tiout_flg/1 -> 2A7_100ms_sys/5(GbISP_2A7Tiout_flg)
  2A7_100ms_sys/1(GeVDP_VcuFalutLvl_enum) -> GeVDP_VcuFalutLvl_enum/1
  2A7_100ms_sys/2(GeVDP_VcuWrkSt_enum) -> GeVDP_VcuWrkSt_enum/1
  2A7_100ms_sys/3(GbVDP_BrkPedSt_flg) -> GbVDP_BrkPedSt_flg/1
  2A7_100ms_sys/4(GbVDP_BrkPedInvld_flg) -> GbVDP_BrkPedInvld_flg/1
  GbVDP_DiagPermit_flg/1 -> 2A7_100ms_sys/6(GbVDP_DiagPermit_flg)
  GbISP_ChkSumMsg2A7Err_flg/1 -> 2A7_100ms_sys/7(GbISP_ChkSumMsg2A7Err_flg)
  GbISP_RcMsg2A7Err_flg/1 -> 2A7_100ms_sys/8(GbISP_RcMsg2A7Err_flg)
  2A7_100ms_sys/5(GbVDP_2A7Tiout_flg) -> GbVDP_2A7Tiout_flg/1
  2A7_100ms_sys/7(GbVDP_2A7RCMsg_flg) -> GbVDP_2A7RCMsg_flg/1
  2A7_100ms_sys/6(GbVDP_2A7ChkSum_flg) -> GbVDP_2A7ChkSum_flg/1

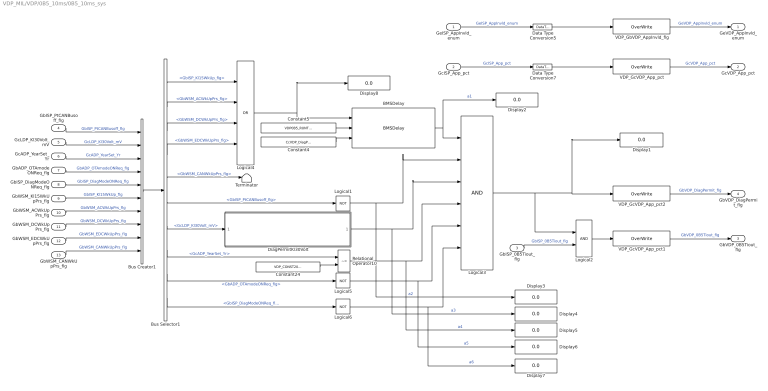
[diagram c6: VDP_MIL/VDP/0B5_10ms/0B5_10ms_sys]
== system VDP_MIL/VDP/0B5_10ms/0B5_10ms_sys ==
  GeISP_AppInvld_enum : Inport
  GcISP_App_pct : Inport  Port=2
  GbISP_0B5Tiout_flg : Inport  Port=3
  GbISP_PtCANBusoff_flg : Inport  Port=4
  GcLDP_Kl30Volt_mV : Inport  Port=5
  GcADP_YearSet_Yr : Inport  Port=6
  GbADP_OTAmodeONReq_flg : Inport  Port=7
  GbISP_DiagModeONReq_flg : Inport  Port=8
  GbWSM_Kl15WkUpPrs_flg : Inport  Port=9
  GbWSM_ACWkUpPrs_flg : Inport  Port=10
  GbWSM_DCWkUpPrs_flg : Inport  Port=11
  GbWSM_EDCWkUpPrs_flg : Inport  Port=12
  GbWSM_CANWkUpPrs_flg : Inport  Port=13
  BMSDelay : AIWAYS_Powertrain_BMS_lib/Debounce & Delay/BMSDelay
  Bus Creator1 : BusCreator  Inputs=10
  Bus Selector1 : BusSelector  OutputSignals=GbISP_Kl15WkUp_flg,GbWSM_ACWkUpPrs_flg,GbWSM_DCWkUpPrs_flg,GbWSM_EDCWkUpPrs_flg,GbWSM_CANWkUpPrs_flg,GbISP_PtCANBusoff_flg,GcLDP_Kl30Volt_mV,GcADP_YearSet_Yr,GbADP_OTAmodeONReq_flg,GbISP_DiagModeONReq_flg
  Constant24 : Constant  Value=VDP_CONST2080_NUMB
  Constant4 : Constant  Value=CcVDP_DiagPermitDelayTi_ms
  Constant5 : Constant  Value=VDP0B5_RUNTIME_MS
  Data Type Conversion5 : DataTypeConversion
  Data Type Conversion7 : DataTypeConversion
  DiagPermitKl30Volt : Subsystem
  Display{1..8} (8 alike) : Display
  Logical1 : Logic  Operator=NOT  OutDataTypeStr=boolean
  Logical2 : Logic  OutDataTypeStr=boolean
  Logical3 : Logic  Inputs=6  OutDataTypeStr=boolean
  Logical4 : Logic  Operator=OR  Inputs=4  OutDataTypeStr=boolean
  Logical5 : Logic  Operator=NOT  OutDataTypeStr=boolean
  Logical6 : Logic  Operator=NOT  OutDataTypeStr=boolean
  Relational Operator10 : RelationalOperator  Operator=~=  OutDataTypeStr=boolean
  Terminator : Terminator
  VDP_GbVDP_AppInvld_flg : AIWAYS_Powertrain_BMS_lib/Signals/OverWrite  OverWrite_Value=CeVDP_AppInvldOvr_enum  OverWrite_flag=CbVDP_AppInvldOvrSwt_flg
  VDP_GcVDP_App_pct : AIWAYS_Powertrain_BMS_lib/Signals/OverWrite  OverWrite_Value=CcVDP_AppOvr_pct  OverWrite_flag=CbVDP_AppOvrSwt_flg
  VDP_GcVDP_App_pct1 : AIWAYS_Powertrain_BMS_lib/Signals/OverWrite  OverWrite_Value=CbVDP_0B5TioutOvr_flg  OverWrite_flag=CbVDP_0B5TioutOvrSwt_flg
  VDP_GcVDP_App_pct2 : AIWAYS_Powertrain_BMS_lib/Signals/OverWrite  OverWrite_Value=CbVDP_DiagPermitOvr_flg  OverWrite_flag=CbVDP_DiagPermitOvrSwt_flg
  GeVDP_AppInvld_enum : Outport
  GcVDP_App_pct : Outport  Port=2
  GbVDP_0B5Tiout_flg : Outport  Port=3
  GbVDP_DiagPermit_flg : Outport  Port=4
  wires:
  GbISP_0B5Tiout_flg/1 -> Logical2/2  "GbISP_0B5Tiout_flg"
  GeISP_AppInvld_enum/1 -> Data Type Conversion5/1  "GeISP_AppInvld_enum"
  GcISP_App_pct/1 -> Data Type Conversion7/1  "GcISP_App_pct"
  Data Type Conversion5/1 -> VDP_GbVDP_AppInvld_flg/1
  VDP_GbVDP_AppInvld_flg/1 -> GeVDP_AppInvld_enum/1  "GeVDP_AppInvld_enum"
  Data Type Conversion7/1 -> VDP_GcVDP_App_pct/1
  VDP_GcVDP_App_pct/1 -> GcVDP_App_pct/1  "GcVDP_App_pct"
  Logical2/1 -> VDP_GcVDP_App_pct1/1
  VDP_GcVDP_App_pct1/1 -> GbVDP_0B5Tiout_flg/1  "GbVDP_0B5Tiout_flg"
  DiagPermitKl30Volt/1(LbVDP_DiagPermitKl30Volt_flg) -> Display4/1, Logical3/3  "a3"
  Bus Creator1/1 -> Bus Selector1/1
  GbISP_PtCANBusoff_flg/1 -> Bus Creator1/1  "GbISP_PtCANBusoff_flg"
  GcLDP_Kl30Volt_mV/1 -> Bus Creator1/2  "GcLDP_Kl30Volt_mV"
  Relational Operator10/1 -> Display5/1, Logical3/4  "a4"
  Bus Selector1/8 -> Relational Operator10/1  "<GcADP_YearSet_Yr>"
  Bus Selector1/7 -> DiagPermitKl30Volt/1(GcLDP_Kl30Volt_mV)  "<GcLDP_Kl30Volt_mV>"
  Logical6/1 -> Display7/1, Logical3/6  "a6"
  BMSDelay/1 -> Display2/1, Logical3/1  "a1"
  Bus Selector1/10 -> Logical6/1  "<GbISP_DiagModeONReq_flg>"
  Bus Selector1/9 -> Logical5/1  "<GbADP_OTAmodeONReq_flg>"
  Constant24/1 -> Relational Operator10/2
  GcADP_YearSet_Yr/1 -> Bus Creator1/3  "GcADP_YearSet_Yr"
  Logical3/1 -> Logical2/1, Display1/1, VDP_GcVDP_App_pct2/1
  Logical1/1 -> Display3/1, Logical3/2  "a2"
  Logical5/1 -> Display6/1, Logical3/5  "a5"
  GbADP_OTAmodeONReq_flg/1 -> Bus Creator1/4  "GbADP_OTAmodeONReq_flg"
  GbISP_DiagModeONReq_flg/1 -> Bus Creator1/5  "GbISP_DiagModeONReq_flg"
  Bus Selector1/6 -> Logical1/1  "<GbISP_PtCANBusoff_flg>"
  VDP_GcVDP_App_pct2/1 -> GbVDP_DiagPermit_flg/1  "GbVDP_DiagPermit_flg"
  Constant5/1 -> BMSDelay/2
  Constant4/1 -> BMSDelay/3
  Bus Selector1/5 -> Terminator/1  "<GbWSM_CANWkUpPrs_flg>"
  Bus Selector1/4 -> Logical4/4  "<GbWSM_EDCWkUpPrs_flg>"
  Bus Selector1/3 -> Logical4/3  "<GbWSM_DCWkUpPrs_flg>"
  Bus Selector1/2 -> Logical4/2  "<GbWSM_ACWkUpPrs_flg>"
  GbWSM_Kl15WkUpPrs_flg/1 -> Bus Creator1/6  "GbISP_Kl15WkUp_flg"
  GbWSM_ACWkUpPrs_flg/1 -> Bus Creator1/7  "GbWSM_ACWkUpPrs_flg"
  GbWSM_DCWkUpPrs_flg/1 -> Bus Creator1/8  "GbWSM_DCWkUpPrs_flg"
  GbWSM_EDCWkUpPrs_flg/1 -> Bus Creator1/9  "GbWSM_EDCWkUpPrs_flg"
  GbWSM_CANWkUpPrs_flg/1 -> Bus Creator1/10  "GbWSM_CANWkUpPrs_flg"
  Bus Selector1/1 -> Logical4/1  "<GbISP_Kl15WkUp_flg>"
  Logical4/1 -> Display8/1, BMSDelay/1

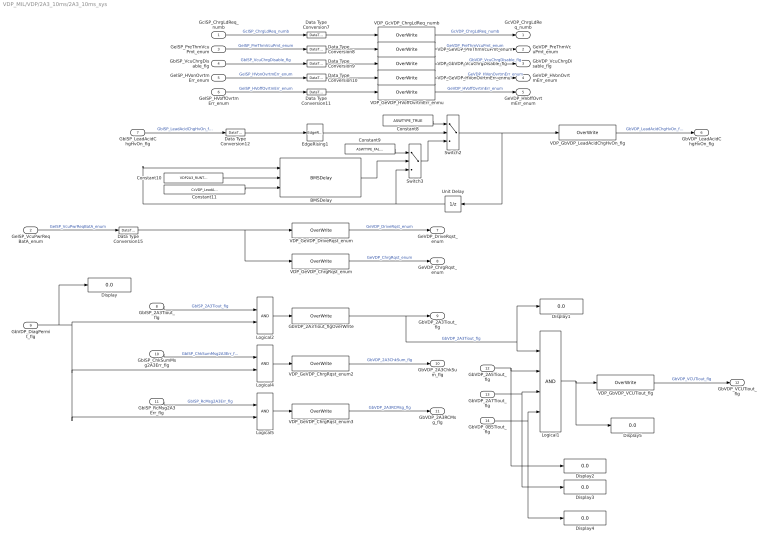
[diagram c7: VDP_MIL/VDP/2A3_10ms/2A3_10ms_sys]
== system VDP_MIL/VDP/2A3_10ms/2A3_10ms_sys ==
  GcISP_ChrgLdReq_numb : Inport
  GeISP_VcuPwrReqBatA_enum : Inport  Port=2
  GeISP_PreThmVcuPmt_enum : Inport  Port=3
  GbISP_VcuChrgDisable_flg : Inport  Port=4
  GeISP_HVonOvrtmErr_enum : Inport  Port=5
  GeISP_HVoffOvrtmErr_enum : Inport  Port=6
  GbISP_LeadAcidChgHvOn_flg : Inport  Port=7
  GbISP_2A3Tiout_flg : Inport  Port=8
  GbVDP_DiagPermit_flg : Inport  Port=9
  GbISP_ChkSumMsg2A3Err_flg : Inport  Port=10
  GbISP_RcMsg2A3Err_flg : Inport  Port=11
  GbVDP_2A5Tiout_flg : Inport  Port=12
  GbVDP_2A7Tiout_flg : Inport  Port=13
  GbVDP_0B5Tiout_flg : Inport  Port=14
  BMSDelay : AIWAYS_Powertrain_BMS_lib/Debounce & Delay/BMSDelay
  Constant10 : Constant  Value=VDP2A3_RUNTIME_MS
  Constant11 : Constant  Value=CcVDP_LeadAcidChgHvOnTi_ms
  Constant8 : Constant  Value=ASWTYPE_TRUE
  Constant9 : Constant  Value=ASWTYPE_FALSE
  Data Type Conversion{7..12,15} (7 alike) : DataTypeConversion
  Display{,1..5} (6 alike) : Display
  EdgeRising1 : AIWAYS_Powertrain_BMS_lib/Logical Operators/EdgeRising
  GbVDP_2A3Tiout_flgOverWrite : AIWAYS_Powertrain_BMS_lib/Signals/OverWrite  OverWrite_Value=CbVDP_2A3TioutOvr_flg  OverWrite_flag=CbVDP_2A3TioutOvrSwt_flg
  Logical1 : Logic  Inputs=4  OutDataTypeStr=boolean
  Logical2 : Logic  OutDataTypeStr=boolean
  Logical4 : Logic  OutDataTypeStr=boolean
  Logical5 : Logic  OutDataTypeStr=boolean
  Switch2 : Switch  Criteria=u2 ~= 0
  Switch3 : Switch  Criteria=u2 ~= 0
  Unit Delay : UnitDelay  SampleTime=-1  StateName=StateName
  VDP_GbVDP_LeadAcidChgHvOn_flg : AIWAYS_Powertrain_BMS_lib/Signals/OverWrite  OverWrite_Value=CbVDP_LeadAcidChgHvOnOvr_flg  OverWrite_flag=CbVDP_LeadAcidChgHvOnOvrSwt_flg
  VDP_GbVDP_VCUTiout_flg : AIWAYS_Powertrain_BMS_lib/Signals/OverWrite  OverWrite_Value=CbVDP_VCUTioutOvr_flg  OverWrite_flag=CbVDP_VCUTioutOvrSwt_flg
  VDP_GbVDP_VcuChrgDisable_flg : AIWAYS_Powertrain_BMS_lib/Signals/OverWrite  OverWrite_Value=CbVDP_VcuChrgDisableOvr_flg  OverWrite_flag=CbVDP_VcuChrgDisableOvrSwt_flg
  VDP_GcVDP_ChrgLdReq_numb : AIWAYS_Powertrain_BMS_lib/Signals/OverWrite  OverWrite_Value=CcVDP_ChrgLdReqOvr_numb  OverWrite_flag=CbVDP_ChrgLdReqOvrSwt_flg
  VDP_GeVDP_ChrgRqst_enum : AIWAYS_Powertrain_BMS_lib/Signals/OverWrite  OverWrite_Value=CeVDP_ChrgRqstOvr_enum  OverWrite_flag=CbVDP_ChrgRqstOvrSwt_flg
  VDP_GeVDP_ChrgRqst_enum2 : AIWAYS_Powertrain_BMS_lib/Signals/OverWrite  OverWrite_Value=CbVDP_2A3ChkSumOvr_flg  OverWrite_flag=CbVDP_2A3ChkSumOvrSwt_flg
  VDP_GeVDP_ChrgRqst_enum3 : AIWAYS_Powertrain_BMS_lib/Signals/OverWrite  OverWrite_Value=CbVDP_2A3RCMsgOvr_flg  OverWrite_flag=CbVDP_2A3RCMsgOvrSwt_flg
  VDP_GeVDP_DriveRqst_enum : AIWAYS_Powertrain_BMS_lib/Signals/OverWrite  OverWrite_Value=CeVDP_DriveRqstOvr_enum  OverWrite_flag=CbVDP_DriveRqstOvrSwt_flg
  VDP_GeVDP_HVoffOvrtmErr_enmu : AIWAYS_Powertrain_BMS_lib/Signals/OverWrite  OverWrite_Value=CeVDP_HVoffOvrtmErrOvr_enum  OverWrite_flag=CbVDP_HVoffOvrtmErrOvrSwt_flg
  VDP_GeVDP_HVonOvrtmErr_enmu : AIWAYS_Powertrain_BMS_lib/Signals/OverWrite  OverWrite_Value=CeVDP_HVonOvrtmErrOvr_enum  OverWrite_flag=CbVDP_HVonOvrtmErrOvrSwt_flg
  VDP_GeVDP_PreThmVcuPmt_enum : AIWAYS_Powertrain_BMS_lib/Signals/OverWrite  OverWrite_Value=CeVDP_PreThmVcuPmtOvr_enum  OverWrite_flag=CbVDP_PreThmVcuPmtOvrSwt_flg
  GcVDP_ChrgLdReq_numb : Outport
  GeVDP_PreThmVcuPmt_enum : Outport  Port=2
  GbVDP_VcuChrgDisable_flg : Outport  Port=3
  GeVDP_HVonOvrtmErr_enum : Outport  Port=4
  GeVDP_HVoffOvrtmErr_enum : Outport  Port=5
  GbVDP_LeadAcidChgHvOn_flg : Outport  Port=6
  GeVDP_DriveRqst_enum : Outport  Port=7
  GeVDP_ChrgRqst_enum : Outport  Port=8
  GbVDP_2A3Tiout_flg : Outport  Port=9
  GbVDP_2A3ChkSum_flg : Outport  Port=10
  GbVDP_2A3RCMsg_flg : Outport  Port=11
  GbVDP_VCUTiout_flg : Outport  Port=12
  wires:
  GbISP_2A3Tiout_flg/1 -> Logical2/1  "GbISP_2A3Tiout_flg"
  GcISP_ChrgLdReq_numb/1 -> Data Type Conversion7/1  "GcISP_ChrgLdReq_numb"
  GeISP_PreThmVcuPmt_enum/1 -> Data Type Conversion8/1  "GeISP_PreThmVcuPmt_enum"
  GbISP_VcuChrgDisable_flg/1 -> Data Type Conversion9/1  "GbISP_VcuChrgDisable_flg"
  GeISP_HVonOvrtmErr_enum/1 -> Data Type Conversion10/1  "GeISP_HVonOvrtmErr_enum"
  GeISP_HVoffOvrtmErr_enum/1 -> Data Type Conversion11/1  "GeISP_HVoffOvrtmErr_enum"
  GbISP_LeadAcidChgHvOn_flg/1 -> Data Type Conversion12/1  "GbISP_LeadAcidChgHvOn_flg"
  VDP_GcVDP_ChrgLdReq_numb/1 -> GcVDP_ChrgLdReq_numb/1  "GcVDP_ChrgLdReq_numb"
  VDP_GeVDP_PreThmVcuPmt_enum/1 -> GeVDP_PreThmVcuPmt_enum/1  "GeVDP_PreThmVcuPmt_enum"
  VDP_GbVDP_VcuChrgDisable_flg/1 -> GbVDP_VcuChrgDisable_flg/1  "GbVDP_VcuChrgDisable_flg"
  VDP_GeVDP_HVonOvrtmErr_enmu/1 -> GeVDP_HVonOvrtmErr_enum/1  "GeVDP_HVonOvrtmErr_enum"
  VDP_GeVDP_HVoffOvrtmErr_enmu/1 -> GeVDP_HVoffOvrtmErr_enum/1  "GeVDP_HVoffOvrtmErr_enum"
  VDP_GbVDP_LeadAcidChgHvOn_flg/1 -> GbVDP_LeadAcidChgHvOn_flg/1  "GbVDP_LeadAcidChgHvOn_flg"
  Data Type Conversion7/1 -> VDP_GcVDP_ChrgLdReq_numb/1
  Data Type Conversion8/1 -> VDP_GeVDP_PreThmVcuPmt_enum/1
  Data Type Conversion9/1 -> VDP_GbVDP_VcuChrgDisable_flg/1
  Data Type Conversion10/1 -> VDP_GeVDP_HVonOvrtmErr_enmu/1
  Data Type Conversion11/1 -> VDP_GeVDP_HVoffOvrtmErr_enmu/1
  Switch2/1 -> Unit Delay/1, VDP_GbVDP_LeadAcidChgHvOn_flg/1
  GeISP_VcuPwrReqBatA_enum/1 -> Data Type Conversion15/1  "GeISP_VcuPwrReqBatA_enum"
  VDP_GeVDP_DriveRqst_enum/1 -> GeVDP_DriveRqst_enum/1  "GeVDP_DriveRqst_enum"
  Data Type Conversion15/1 -> VDP_GeVDP_DriveRqst_enum/1, VDP_GeVDP_ChrgRqst_enum/1
  VDP_GeVDP_ChrgRqst_enum/1 -> GeVDP_ChrgRqst_enum/1  "GeVDP_ChrgRqst_enum"
  GbVDP_DiagPermit_flg/1 -> Display/1, Logical2/2, Logical5/2, Logical4/2
  Logical2/1 -> GbVDP_2A3Tiout_flgOverWrite/1
  GbISP_ChkSumMsg2A3Err_flg/1 -> Logical4/1  "GbISP_ChkSumMsg2A3Err_flg"
  Logical4/1 -> VDP_GeVDP_ChrgRqst_enum2/1
  GbISP_RcMsg2A3Err_flg/1 -> Logical5/1  "GbISP_RcMsg2A3Err_flg"
  Logical5/1 -> VDP_GeVDP_ChrgRqst_enum3/1
  VDP_GeVDP_ChrgRqst_enum2/1 -> GbVDP_2A3ChkSum_flg/1  "GbVDP_2A3ChkSum_flg"
  VDP_GeVDP_ChrgRqst_enum3/1 -> GbVDP_2A3RCMsg_flg/1  "GbVDP_2A3RCMsg_flg"
  GbVDP_2A3Tiout_flgOverWrite/1 -> Display1/1, Logical1/1, GbVDP_2A3Tiout_flg/1  "GbVDP_2A3Tiout_flg"
  GbVDP_2A5Tiout_flg/1 -> Display2/1, Logical1/2
  GbVDP_2A7Tiout_flg/1 -> Display3/1, Logical1/3
  Logical1/1 -> Display5/1, VDP_GbVDP_VCUTiout_flg/1
  VDP_GbVDP_VCUTiout_flg/1 -> GbVDP_VCUTiout_flg/1  "GbVDP_VCUTiout_flg"
  Constant8/1 -> Switch2/1
  Data Type Conversion12/1 -> EdgeRising1/1
  EdgeRising1/1 -> Switch2/2
  Unit Delay/1 -> BMSDelay/1, Switch3/3
  Switch3/1 -> Switch2/3
  BMSDelay/1 -> Switch3/2
  Constant9/1 -> Switch3/1
  Constant10/1 -> BMSDelay/2
  Constant11/1 -> BMSDelay/3
  GbVDP_0B5Tiout_flg/1 -> Display4/1, Logical1/4

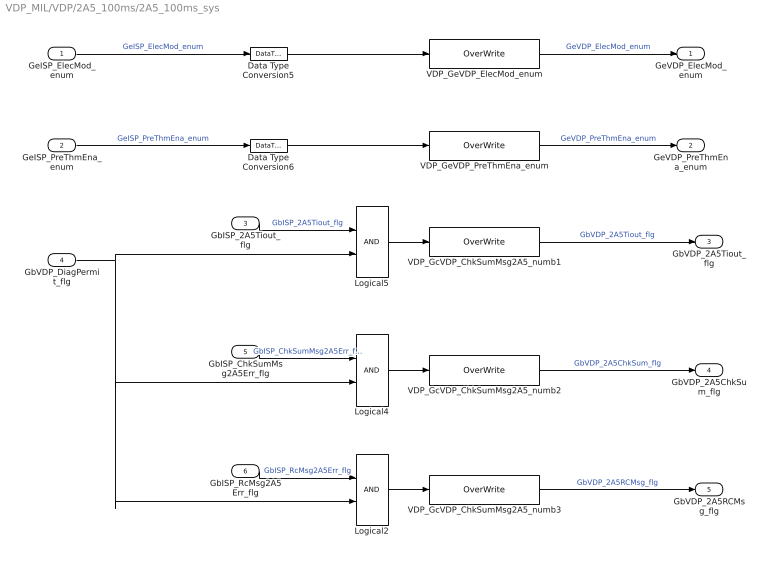
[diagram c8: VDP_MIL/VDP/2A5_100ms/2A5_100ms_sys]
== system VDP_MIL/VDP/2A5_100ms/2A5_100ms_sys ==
  GeISP_ElecMod_enum : Inport
  GeISP_PreThmEna_enum : Inport  Port=2
  GbISP_2A5Tiout_flg : Inport  Port=3
  GbVDP_DiagPermit_flg : Inport  Port=4
  GbISP_ChkSumMsg2A5Err_flg : Inport  Port=5
  GbISP_RcMsg2A5Err_flg : Inport  Port=6
  Data Type Conversion5 : DataTypeConversion
  Data Type Conversion6 : DataTypeConversion
  Logical2 : Logic  OutDataTypeStr=boolean
  Logical4 : Logic  OutDataTypeStr=boolean
  Logical5 : Logic  OutDataTypeStr=boolean
  VDP_GcVDP_ChkSumMsg2A5_numb1 : AIWAYS_Powertrain_BMS_lib/Signals/OverWrite  OverWrite_Value=CbVDP_2A5TioutOvr_flg  OverWrite_flag=CbVDP_2A5TioutOvrSwt_flg
  VDP_GcVDP_ChkSumMsg2A5_numb2 : AIWAYS_Powertrain_BMS_lib/Signals/OverWrite  OverWrite_Value=CbVDP_2A5ChkSumOvr_flg  OverWrite_flag=CbVDP_2A5ChkSumOvrSwt_flg
  VDP_GcVDP_ChkSumMsg2A5_numb3 : AIWAYS_Powertrain_BMS_lib/Signals/OverWrite  OverWrite_Value=CbVDP_2A5RCMsgOvr_flg  OverWrite_flag=CbVDP_2A5RCMsgOvrSwt_flg
  VDP_GeVDP_ElecMod_enum : AIWAYS_Powertrain_BMS_lib/Signals/OverWrite  OverWrite_Value=CeVDP_ElecModOvr_enum  OverWrite_flag=CbVDP_ElecModOvrSwt_flg
  VDP_GeVDP_PreThmEna_enum : AIWAYS_Powertrain_BMS_lib/Signals/OverWrite  OverWrite_Value=CeVDP_PreThmEnaOvr_enum  OverWrite_flag=CbVDP_PreThmEnaOvrSwt_flg
  GeVDP_ElecMod_enum : Outport
  GeVDP_PreThmEna_enum : Outport  Port=2
  GbVDP_2A5Tiout_flg : Outport  Port=3
  GbVDP_2A5ChkSum_flg : Outport  Port=4
  GbVDP_2A5RCMsg_flg : Outport  Port=5
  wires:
  GeISP_ElecMod_enum/1 -> Data Type Conversion5/1  "GeISP_ElecMod_enum"
  GeISP_PreThmEna_enum/1 -> Data Type Conversion6/1  "GeISP_PreThmEna_enum"
  GbISP_2A5Tiout_flg/1 -> Logical5/1  "GbISP_2A5Tiout_flg"
  VDP_GeVDP_ElecMod_enum/1 -> GeVDP_ElecMod_enum/1  "GeVDP_ElecMod_enum"
  VDP_GeVDP_PreThmEna_enum/1 -> GeVDP_PreThmEna_enum/1  "GeVDP_PreThmEna_enum"
  Logical5/1 -> VDP_GcVDP_ChkSumMsg2A5_numb1/1
  GbISP_RcMsg2A5Err_flg/1 -> Logical2/1  "GbISP_RcMsg2A5Err_flg"
  Logical2/1 -> VDP_GcVDP_ChkSumMsg2A5_numb3/1
  Logical4/1 -> VDP_GcVDP_ChkSumMsg2A5_numb2/1
  GbVDP_DiagPermit_flg/1 -> Logical2/2, Logical4/2, Logical5/2
  GbISP_ChkSumMsg2A5Err_flg/1 -> Logical4/1  "GbISP_ChkSumMsg2A5Err_flg"
  VDP_GcVDP_ChkSumMsg2A5_numb1/1 -> GbVDP_2A5Tiout_flg/1  "GbVDP_2A5Tiout_flg"
  VDP_GcVDP_ChkSumMsg2A5_numb2/1 -> GbVDP_2A5ChkSum_flg/1  "GbVDP_2A5ChkSum_flg"
  VDP_GcVDP_ChkSumMsg2A5_numb3/1 -> GbVDP_2A5RCMsg_flg/1  "GbVDP_2A5RCMsg_flg"
  Data Type Conversion5/1 -> VDP_GeVDP_ElecMod_enum/1
  Data Type Conversion6/1 -> VDP_GeVDP_PreThmEna_enum/1

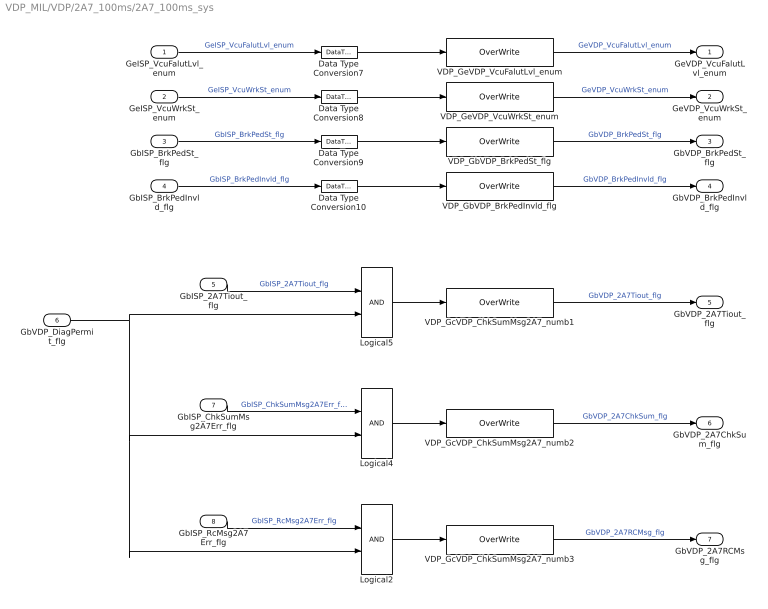
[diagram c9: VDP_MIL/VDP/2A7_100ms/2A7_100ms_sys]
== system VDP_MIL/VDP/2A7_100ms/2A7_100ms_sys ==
  GeISP_VcuFalutLvl_enum : Inport
  GeISP_VcuWrkSt_enum : Inport  Port=2
  GbISP_BrkPedSt_flg : Inport  Port=3
  GbISP_BrkPedInvld_flg : Inport  Port=4
  GbISP_2A7Tiout_flg : Inport  Port=5
  GbVDP_DiagPermit_flg : Inport  Port=6
  GbISP_ChkSumMsg2A7Err_flg : Inport  Port=7
  GbISP_RcMsg2A7Err_flg : Inport  Port=8
  Data Type Conversion{7..10} (4 alike) : DataTypeConversion
  Logical2 : Logic  OutDataTypeStr=boolean
  Logical4 : Logic  OutDataTypeStr=boolean
  Logical5 : Logic  OutDataTypeStr=boolean
  VDP_GbVDP_BrkPedInvld_flg : AIWAYS_Powertrain_BMS_lib/Signals/OverWrite  OverWrite_Value=CbVDP_BrkPedInvldOvr_flg  OverWrite_flag=CbVDP_BrkPedInvldOvrSwt_flg
  VDP_GbVDP_BrkPedSt_flg : AIWAYS_Powertrain_BMS_lib/Signals/OverWrite  OverWrite_Value=CbVDP_BrkPedStOvr_flg  OverWrite_flag=CbVDP_BrkPedStOvrSwt_flg
  VDP_GcVDP_ChkSumMsg2A7_numb1 : AIWAYS_Powertrain_BMS_lib/Signals/OverWrite  OverWrite_Value=CbVDP_2A7TioutOvr_flg  OverWrite_flag=CbVDP_2A7TioutOvrSwt_flg
  VDP_GcVDP_ChkSumMsg2A7_numb2 : AIWAYS_Powertrain_BMS_lib/Signals/OverWrite  OverWrite_Value=CbVDP_2A7ChkSumOvr_flg  OverWrite_flag=CbVDP_2A7ChkSumOvrSwt_flg
  VDP_GcVDP_ChkSumMsg2A7_numb3 : AIWAYS_Powertrain_BMS_lib/Signals/OverWrite  OverWrite_Value=CbVDP_2A7RCMsgOvr_flg  OverWrite_flag=CbVDP_2A7RCMsgOvrSwt_flg
  VDP_GeVDP_VcuFalutLvl_enum : AIWAYS_Powertrain_BMS_lib/Signals/OverWrite  OverWrite_Value=CeVDP_VcuFalutLvlOvr_enum  OverWrite_flag=CbVDP_VcuFalutLvlOvrSwt_flg
  VDP_GeVDP_VcuWrkSt_enum : AIWAYS_Powertrain_BMS_lib/Signals/OverWrite  OverWrite_Value=CeVDP_VcuWrkStOvr_enum  OverWrite_flag=CbVDP_VcuWrkStOvrSwt_flg
  GeVDP_VcuFalutLvl_enum : Outport
  GeVDP_VcuWrkSt_enum : Outport  Port=2
  GbVDP_BrkPedSt_flg : Outport  Port=3
  GbVDP_BrkPedInvld_flg : Outport  Port=4
  GbVDP_2A7Tiout_flg : Outport  Port=5
  GbVDP_2A7ChkSum_flg : Outport  Port=6
  GbVDP_2A7RCMsg_flg : Outport  Port=7
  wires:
  GeISP_VcuFalutLvl_enum/1 -> Data Type Conversion7/1  "GeISP_VcuFalutLvl_enum"
  GeISP_VcuWrkSt_enum/1 -> Data Type Conversion8/1  "GeISP_VcuWrkSt_enum"
  GbISP_BrkPedSt_flg/1 -> Data Type Conversion9/1  "GbISP_BrkPedSt_flg"
  GbISP_BrkPedInvld_flg/1 -> Data Type Conversion10/1  "GbISP_BrkPedInvld_flg"
  GbISP_2A7Tiout_flg/1 -> Logical5/1  "GbISP_2A7Tiout_flg"
  VDP_GeVDP_VcuFalutLvl_enum/1 -> GeVDP_VcuFalutLvl_enum/1  "GeVDP_VcuFalutLvl_enum"
  VDP_GeVDP_VcuWrkSt_enum/1 -> GeVDP_VcuWrkSt_enum/1  "GeVDP_VcuWrkSt_enum"
  VDP_GbVDP_BrkPedSt_flg/1 -> GbVDP_BrkPedSt_flg/1  "GbVDP_BrkPedSt_flg"
  VDP_GbVDP_BrkPedInvld_flg/1 -> GbVDP_BrkPedInvld_flg/1  "GbVDP_BrkPedInvld_flg"
  Data Type Conversion7/1 -> VDP_GeVDP_VcuFalutLvl_enum/1
  Data Type Conversion8/1 -> VDP_GeVDP_VcuWrkSt_enum/1
  Data Type Conversion9/1 -> VDP_GbVDP_BrkPedSt_flg/1
  Data Type Conversion10/1 -> VDP_GbVDP_BrkPedInvld_flg/1
  Logical5/1 -> VDP_GcVDP_ChkSumMsg2A7_numb1/1
  GbVDP_DiagPermit_flg/1 -> Logical5/2, Logical4/2, Logical2/2
  Logical4/1 -> VDP_GcVDP_ChkSumMsg2A7_numb2/1
  GbISP_ChkSumMsg2A7Err_flg/1 -> Logical4/1  "GbISP_ChkSumMsg2A7Err_flg"
  GbISP_RcMsg2A7Err_flg/1 -> Logical2/1  "GbISP_RcMsg2A7Err_flg"
  Logical2/1 -> VDP_GcVDP_ChkSumMsg2A7_numb3/1
  VDP_GcVDP_ChkSumMsg2A7_numb1/1 -> GbVDP_2A7Tiout_flg/1  "GbVDP_2A7Tiout_flg"
  VDP_GcVDP_ChkSumMsg2A7_numb2/1 -> GbVDP_2A7ChkSum_flg/1  "GbVDP_2A7ChkSum_flg"
  VDP_GcVDP_ChkSumMsg2A7_numb3/1 -> GbVDP_2A7RCMsg_flg/1  "GbVDP_2A7RCMsg_flg"

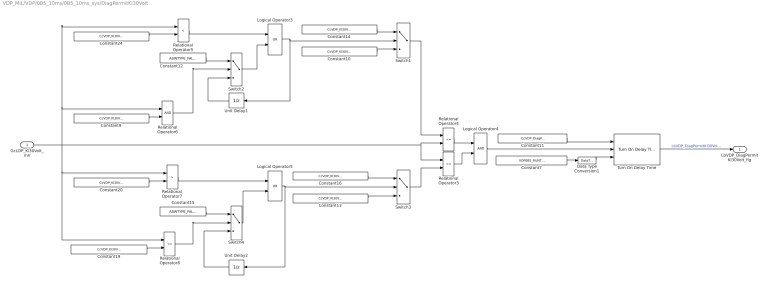
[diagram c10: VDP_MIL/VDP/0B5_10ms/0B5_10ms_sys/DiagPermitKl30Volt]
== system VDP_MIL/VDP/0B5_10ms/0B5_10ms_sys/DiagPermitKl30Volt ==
  GcLDP_Kl30Volt_mV : Inport
  Constant10 : Constant  Value=CcVDP_Kl30VoltNorm2Under_mV
  Constant11 : Constant  Value=CcVDP_DiagPermitDelayTi_ms
  Constant12 : Constant  Value=ASWTYPE_FALSE
  Constant13 : Constant  Value=CcVDP_Kl30VoltNorm2Over_mV
  Constant14 : Constant  Value=CcVDP_Kl30VoltUnder2Norm_mV
  Constant15 : Constant  Value=ASWTYPE_FALSE
  Constant16 : Constant  Value=CcVDP_Kl30VoltOver2Norm_mV
  Constant19 : Constant  Value=CcVDP_Kl30VoltOver2Norm_mV
  Constant20 : Constant  Value=CcVDP_Kl30VoltNorm2Over_mV
  Constant24 : Constant  Value=CcVDP_Kl30VoltNorm2Under_mV
  Constant7 : Constant  Value=VDP0B5_RUNTIME_MS
  Constant9 : Constant  Value=CcVDP_Kl30VoltUnder2Norm_mV
  Data Type Conversion1 : DataTypeConversion
  Logical Operator3 : Logic  Operator=OR  AllPortsSameDT=off  OutDataTypeStr=boolean
  Logical Operator4 : Logic  AllPortsSameDT=off  OutDataTypeStr=boolean
  Logical Operator5 : Logic  Operator=OR  AllPortsSameDT=off  OutDataTypeStr=boolean
  Relational Operator3 : RelationalOperator  Operator=<=  OutDataTypeStr=boolean
  Relational Operator4 : RelationalOperator  Operator=<=  OutDataTypeStr=boolean
  Relational Operator5 : RelationalOperator  Operator=<  OutDataTypeStr=boolean
  Relational Operator6 : RelationalOperator  OutDataTypeStr=boolean
  Relational Operator7 : RelationalOperator  Operator=>  OutDataTypeStr=boolean
  Relational Operator8 : RelationalOperator  Operator=<=  OutDataTypeStr=boolean
  Switch{1..4} (4 alike) : Switch  Criteria=u2 ~= 0  Threshold=1  RndMeth=Zero
  Turn On Delay Time : AIWAYS_Powertrain_BMS_lib/Delay Blocks/Turn On Delay Time
  Unit Delay1 : UnitDelay  SampleTime=-1  StateName=StateName
  Unit Delay2 : UnitDelay  SampleTime=-1  StateName=StateName
  LbVDP_DiagPermitKl30Volt_flg : Outport
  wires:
  Constant9/1 -> Relational Operator6/2
  Switch2/1 -> Logical Operator3/2
  Constant12/1 -> Switch2/1
  Relational Operator6/1 -> Switch2/2
  Relational Operator3/1 -> Logical Operator4/2
  Logical Operator3/1 -> Unit Delay1/1, Switch1/2
  Relational Operator5/1 -> Logical Operator3/1
  Constant14/1 -> Switch1/1
  Unit Delay1/1 -> Switch2/3
  Relational Operator4/1 -> Logical Operator4/1
  Switch3/1 -> Relational Operator3/2
  Constant10/1 -> Switch1/3
  Constant24/1 -> Relational Operator5/2
  Switch1/1 -> Relational Operator4/1
  Logical Operator4/1 -> Turn On Delay Time/2
  Constant7/1 -> Data Type Conversion1/1
  Constant11/1 -> Turn On Delay Time/1
  Constant20/1 -> Relational Operator7/2
  Constant13/1 -> Switch3/3
  Unit Delay2/1 -> Switch4/3
  Constant16/1 -> Switch3/1
  Relational Operator7/1 -> Logical Operator5/1
  Logical Operator5/1 -> Unit Delay2/1, Switch3/2
  Relational Operator8/1 -> Switch4/2
  GcLDP_Kl30Volt_mV/1 -> Relational Operator8/1, Relational Operator7/1, Relational Operator4/2, Relational Operator3/1, Relational Operator6/1, Relational Operator5/1
  Constant15/1 -> Switch4/1
  Switch4/1 -> Logical Operator5/2
  Constant19/1 -> Relational Operator8/2
  Turn On Delay Time/1 -> LbVDP_DiagPermitKl30Volt_flg/1  "LbVDP_DiagPermitKl30Volt_flg"
  Data Type Conversion1/1 -> Turn On Delay Time/3

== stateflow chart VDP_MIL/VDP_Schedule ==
  (default) -> (junction 50)
  (junction 50) -> (junction 13) : { VDP_0B5_10ms; VDP_2A3_10ms; }
  (junction 13) -> (junction 150) : { TimeCounter100ms ++; }
  (junction 150) -> (junction 503) : [TimeCounter100ms >= Const100ms]
  (junction 150) -> (junction 505)
  (junction 503) -> (junction 505) : {VDP_2A5_100ms; VDP_2A7_100ms; TimeCounter100ms = 0; }
  data: Const100ms constant uint8 =10; TimeCounter100ms local uint8
  events: output FUNCTION_CALL_EVENT; output FUNCTION_CALL_EVENT; output FUNCTION_CALL_EVENT; output FUNCTION_CALL_EVENT
